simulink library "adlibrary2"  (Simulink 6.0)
settings: Solver=ode45  StartTime=0.0  StopTime=10.0  RelTol=1e-3
undefined symbols (not defined in the file or in its folder): adlibrary2, ADM, Bit, DDR, Generation, II, Location, Lower, SDRAM, SRAM, Width, XP, XPL, XRC, ZBT
libraries: xbsIndex_r3 x581, adlibrary2 x2
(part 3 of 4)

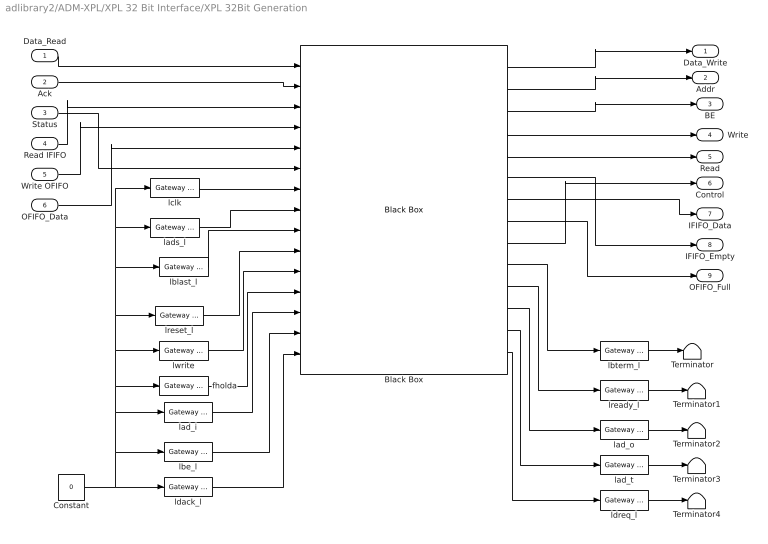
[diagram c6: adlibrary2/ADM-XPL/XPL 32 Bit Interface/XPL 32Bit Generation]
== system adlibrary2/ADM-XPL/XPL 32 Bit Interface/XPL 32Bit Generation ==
  Data_Read : Inport  Port=1  LatchInput=off
  Ack : Inport  Port=2  LatchInput=off
  Status : Inport  Port=3  LatchInput=off
  Read IFIFO : Inport  Port=4  LatchInput=off
  Write OFIFO : Inport  Port=5  LatchInput=off
  OFIFO_Data : Inport  Port=6  LatchInput=off
  Black Box : xbsIndex_r3/Black Box  init_code=lbif32_xpl_config  sim_method=Inactive  show_param=on
  Constant : Constant  Value=0
  Terminator{,1..4} (5 alike) : Terminator
  fholda : xbsIndex_r3/Gateway In  arith_type=Boolean  n_bits=8  bin_pt=6  quantization=Truncate  overflow=Wrap  period=1  timing_constraint=None  locs_specified=off  LOCs={}  needs_fixed_name=off  dbl_ovrd=off  show_param=off
  lad_i : xbsIndex_r3/Gateway In  arith_type=Unsigned  n_bits=64  bin_pt=0  quantization=Truncate  overflow=Wrap  period=1  timing_constraint=None  locs_specified=off  LOCs={}  needs_fixed_name=off  dbl_ovrd=off  show_param=off
  lad_o : xbsIndex_r3/Gateway Out  hdl_port=on  timing_constraint=None  locs_specified=off  LOCs={}  needs_fixed_name=off  show_param=off
  lad_t : xbsIndex_r3/Gateway Out  hdl_port=on  timing_constraint=None  locs_specified=off  LOCs={}  needs_fixed_name=off  show_param=off
  lads_l : xbsIndex_r3/Gateway In  arith_type=Boolean  n_bits=8  bin_pt=6  quantization=Truncate  overflow=Wrap  period=1  timing_constraint=None  locs_specified=off  LOCs={}  needs_fixed_name=off  dbl_ovrd=off  show_param=off
  lbe_l : xbsIndex_r3/Gateway In  arith_type=Unsigned  n_bits=8  bin_pt=0  quantization=Truncate  overflow=Wrap  period=1  timing_constraint=None  locs_specified=off  LOCs={}  needs_fixed_name=off  dbl_ovrd=off  show_param=off
  lblast_l : xbsIndex_r3/Gateway In  arith_type=Boolean  n_bits=8  bin_pt=6  quantization=Truncate  overflow=Wrap  period=1  timing_constraint=None  locs_specified=off  LOCs={}  needs_fixed_name=off  dbl_ovrd=off  show_param=off
  lbterm_l : xbsIndex_r3/Gateway Out  hdl_port=on  timing_constraint=None  locs_specified=off  LOCs={}  needs_fixed_name=off  show_param=off
  lclk : xbsIndex_r3/Gateway In  arith_type=Boolean  n_bits=8  bin_pt=6  quantization=Truncate  overflow=Wrap  period=1  timing_constraint=None  locs_specified=off  LOCs={}  needs_fixed_name=off  dbl_ovrd=off  show_param=off
  ldack_l : xbsIndex_r3/Gateway In  arith_type=Unsigned  n_bits=2  bin_pt=0  quantization=Truncate  overflow=Wrap  period=1  timing_constraint=None  locs_specified=off  LOCs={}  needs_fixed_name=off  dbl_ovrd=off  show_param=off
  ldreq_l : xbsIndex_r3/Gateway Out  hdl_port=on  timing_constraint=None  locs_specified=off  LOCs={}  needs_fixed_name=off  show_param=off
  lready_l : xbsIndex_r3/Gateway Out  hdl_port=on  timing_constraint=None  locs_specified=off  LOCs={}  needs_fixed_name=off  show_param=off
  lreset_l : xbsIndex_r3/Gateway In  arith_type=Boolean  n_bits=8  bin_pt=6  quantization=Truncate  overflow=Wrap  period=1  timing_constraint=None  locs_specified=off  LOCs={}  needs_fixed_name=off  dbl_ovrd=off  show_param=off
  lwrite : xbsIndex_r3/Gateway In  arith_type=Boolean  n_bits=8  bin_pt=6  quantization=Truncate  overflow=Wrap  period=1  timing_constraint=None  locs_specified=off  LOCs={}  needs_fixed_name=off  dbl_ovrd=off  show_param=off
  Data_Write : Outport
  Addr : Outport  Port=2
  BE : Outport  Port=3
  Write : Outport  Port=4
  Read : Outport  Port=5
  Control : Outport  Port=6
  IFIFO_Data : Outport  Port=7
  IFIFO_Empty : Outport  Port=8
  OFIFO_Full : Outport  Port=9
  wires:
  ldreq_l/1 -> Terminator4/1
  lad_t/1 -> Terminator3/1
  lad_o/1 -> Terminator2/1
  lready_l/1 -> Terminator1/1
  lbterm_l/1 -> Terminator/1
  Constant/1 -> lbe_l/1, lad_i/1, fholda/1, lwrite/1, lreset_l/1, lblast_l/1, lads_l/1, lclk/1, ldack_l/1
  ldack_l/1 -> Black Box/15
  lad_i/1 -> Black Box/13
  fholda/1 -> Black Box/12
  lwrite/1 -> Black Box/11
  lreset_l/1 -> Black Box/10
  lblast_l/1 -> Black Box/9
  lads_l/1 -> Black Box/8
  lclk/1 -> Black Box/7
  OFIFO_Data/1 -> Black Box/5
  Write OFIFO/1 -> Black Box/4
  Read IFIFO/1 -> Black Box/3
  Status/1 -> Black Box/6
  Ack/1 -> Black Box/2
  Data_Read/1 -> Black Box/1
  lbe_l/1 -> Black Box/14
  Black Box/1 -> Data_Write/1
  Black Box/2 -> Addr/1
  Black Box/3 -> BE/1
  Black Box/4 -> Write/1
  Black Box/5 -> Read/1
  Black Box/6 -> IFIFO_Empty/1
  Black Box/7 -> IFIFO_Data/1
  Black Box/8 -> OFIFO_Full/1
  Black Box/9 -> Control/1
  Black Box/10 -> lbterm_l/1
  Black Box/11 -> lready_l/1
  Black Box/12 -> lad_o/1
  Black Box/13 -> lad_t/1
  Black Box/14 -> ldreq_l/1

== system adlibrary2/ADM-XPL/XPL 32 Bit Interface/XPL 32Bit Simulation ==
  Data_Read : Inport  Port=1  LatchInput=off
  Ack : Inport  Port=2  LatchInput=off
  Status : Inport  Port=3  LatchInput=off
  Read IFIFO : Inport  Port=4  LatchInput=off
  Write OFIFO : Inport  Port=5  LatchInput=off
  OFIFO_Data : Inport  Port=6  LatchInput=off
  Disregard Subsystem : xbsIndex_r3/Disregard Subsystem  Tag=discardX
  Gateway Out{,1..5} (6 alike) : xbsIndex_r3/Gateway Out  hdl_port=off  timing_constraint=None  locs_specified=off  LOCs={}  needs_fixed_name=off  show_param=off
  S-Function : S-Function  FunctionName=lbif_plx32  Parameters=program,clock_ratio
  Subsystem : Subsystem
  Data_Write : Outport
  Addr : Outport  Port=2
  BE : Outport  Port=3
  Write : Outport  Port=4
  Read : Outport  Port=5
  Control : Outport  Port=6
  IFIFO_Data : Outport  Port=7
  IFIFO_Empty : Outport  Port=8
  OFIFO_Full : Outport  Port=9
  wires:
  Gateway Out5/1 -> S-Function/6
  Gateway Out4/1 -> S-Function/5
  Gateway Out3/1 -> S-Function/4
  Gateway Out2/1 -> S-Function/3
  Gateway Out1/1 -> S-Function/2
  Gateway Out/1 -> S-Function/1
  OFIFO_Data/1 -> Gateway Out5/1
  Write OFIFO/1 -> Gateway Out4/1
  Read IFIFO/1 -> Gateway Out3/1
  Status/1 -> Gateway Out2/1
  Ack/1 -> Gateway Out1/1
  Data_Read/1 -> Gateway Out/1
  S-Function/1 -> Subsystem/1(In1)
  S-Function/2 -> Subsystem/2(In2)
  S-Function/3 -> Subsystem/3(In9)
  S-Function/4 -> Subsystem/4(In3)
  S-Function/5 -> Subsystem/5(In4)
  S-Function/6 -> Subsystem/6(In5)
  S-Function/7 -> Subsystem/7(In6)
  S-Function/8 -> Subsystem/8(In7)
  Subsystem/1(Out1) -> Data_Write/1
  Subsystem/2(Out2) -> Addr/1
  Subsystem/9(Out8) -> OFIFO_Full/1
  Subsystem/8(Out7) -> IFIFO_Empty/1
  Subsystem/7(Out6) -> IFIFO_Data/1
  Subsystem/6(Out5) -> Control/1
  Subsystem/5(Out4) -> Read/1
  Subsystem/4(Out3) -> Write/1
  Subsystem/3(Out9) -> BE/1
  S-Function/9 -> Subsystem/9(In8)

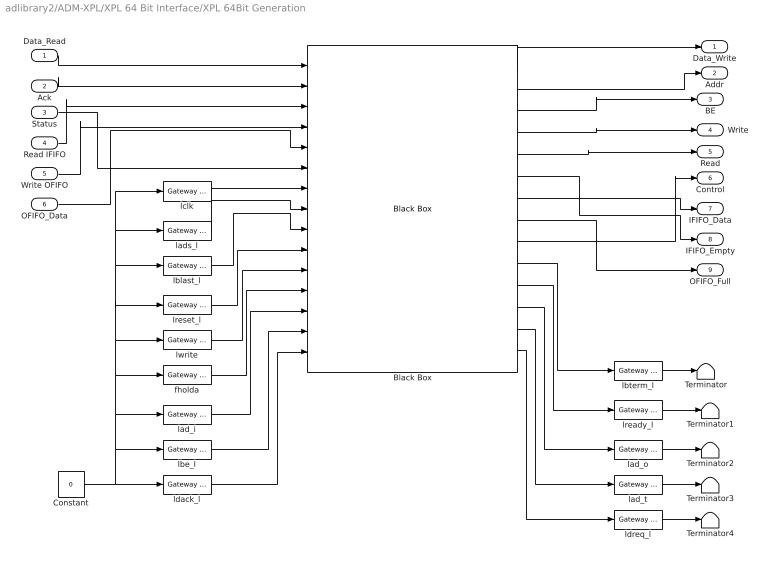
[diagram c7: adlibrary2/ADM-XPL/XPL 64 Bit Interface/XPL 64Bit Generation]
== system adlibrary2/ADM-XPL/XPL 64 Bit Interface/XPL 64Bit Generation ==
  Data_Read : Inport  Port=1  LatchInput=off
  Ack : Inport  Port=2  LatchInput=off
  Status : Inport  Port=3  LatchInput=off
  Read IFIFO : Inport  Port=4  LatchInput=off
  Write OFIFO : Inport  Port=5  LatchInput=off
  OFIFO_Data : Inport  Port=6  LatchInput=off
  Black Box : xbsIndex_r3/Black Box  init_code=lbif64_xpl_config  sim_method=Inactive  show_param=on
  Constant : Constant  Value=0
  Terminator{,1..4} (5 alike) : Terminator
  fholda : xbsIndex_r3/Gateway In  arith_type=Boolean  n_bits=8  bin_pt=6  quantization=Truncate  overflow=Wrap  period=1  timing_constraint=None  locs_specified=off  LOCs={}  needs_fixed_name=off  dbl_ovrd=off  show_param=off
  lad_i : xbsIndex_r3/Gateway In  arith_type=Unsigned  n_bits=64  bin_pt=0  quantization=Truncate  overflow=Wrap  period=1  timing_constraint=None  locs_specified=off  LOCs={}  needs_fixed_name=off  dbl_ovrd=off  show_param=off
  lad_o : xbsIndex_r3/Gateway Out  hdl_port=on  timing_constraint=None  locs_specified=off  LOCs={}  needs_fixed_name=off  show_param=off
  lad_t : xbsIndex_r3/Gateway Out  hdl_port=on  timing_constraint=None  locs_specified=off  LOCs={}  needs_fixed_name=off  show_param=off
  lads_l : xbsIndex_r3/Gateway In  arith_type=Boolean  n_bits=8  bin_pt=6  quantization=Truncate  overflow=Wrap  period=1  timing_constraint=None  locs_specified=off  LOCs={}  needs_fixed_name=off  dbl_ovrd=off  show_param=off
  lbe_l : xbsIndex_r3/Gateway In  arith_type=Unsigned  n_bits=8  bin_pt=0  quantization=Truncate  overflow=Wrap  period=1  timing_constraint=None  locs_specified=off  LOCs={}  needs_fixed_name=off  dbl_ovrd=off  show_param=off
  lblast_l : xbsIndex_r3/Gateway In  arith_type=Boolean  n_bits=8  bin_pt=6  quantization=Truncate  overflow=Wrap  period=1  timing_constraint=None  locs_specified=off  LOCs={}  needs_fixed_name=off  dbl_ovrd=off  show_param=off
  lbterm_l : xbsIndex_r3/Gateway Out  hdl_port=on  timing_constraint=None  locs_specified=off  LOCs={}  needs_fixed_name=off  show_param=off
  lclk : xbsIndex_r3/Gateway In  arith_type=Boolean  n_bits=8  bin_pt=6  quantization=Truncate  overflow=Wrap  period=1  timing_constraint=None  locs_specified=off  LOCs={}  needs_fixed_name=off  dbl_ovrd=off  show_param=off
  ldack_l : xbsIndex_r3/Gateway In  arith_type=Unsigned  n_bits=2  bin_pt=0  quantization=Truncate  overflow=Wrap  period=1  timing_constraint=None  locs_specified=off  LOCs={}  needs_fixed_name=off  dbl_ovrd=off  show_param=off
  ldreq_l : xbsIndex_r3/Gateway Out  hdl_port=on  timing_constraint=None  locs_specified=off  LOCs={}  needs_fixed_name=off  show_param=off
  lready_l : xbsIndex_r3/Gateway Out  hdl_port=on  timing_constraint=None  locs_specified=off  LOCs={}  needs_fixed_name=off  show_param=off
  lreset_l : xbsIndex_r3/Gateway In  arith_type=Boolean  n_bits=8  bin_pt=6  quantization=Truncate  overflow=Wrap  period=1  timing_constraint=None  locs_specified=off  LOCs={}  needs_fixed_name=off  dbl_ovrd=off  show_param=off
  lwrite : xbsIndex_r3/Gateway In  arith_type=Boolean  n_bits=8  bin_pt=6  quantization=Truncate  overflow=Wrap  period=1  timing_constraint=None  locs_specified=off  LOCs={}  needs_fixed_name=off  dbl_ovrd=off  show_param=off
  Data_Write : Outport
  Addr : Outport  Port=2
  BE : Outport  Port=3
  Write : Outport  Port=4
  Read : Outport  Port=5
  Control : Outport  Port=6
  IFIFO_Data : Outport  Port=7
  IFIFO_Empty : Outport  Port=8
  OFIFO_Full : Outport  Port=9
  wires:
  lbe_l/1 -> Black Box/14
  Data_Read/1 -> Black Box/1
  Ack/1 -> Black Box/2
  Status/1 -> Black Box/6
  Read IFIFO/1 -> Black Box/3
  Write OFIFO/1 -> Black Box/4
  OFIFO_Data/1 -> Black Box/5
  Black Box/1 -> Data_Write/1
  Black Box/2 -> Addr/1
  lclk/1 -> Black Box/7
  lads_l/1 -> Black Box/8
  lblast_l/1 -> Black Box/9
  lreset_l/1 -> Black Box/10
  lwrite/1 -> Black Box/11
  fholda/1 -> Black Box/12
  lad_i/1 -> Black Box/13
  ldack_l/1 -> Black Box/15
  Constant/1 -> ldack_l/1, lclk/1, lads_l/1, lblast_l/1, lreset_l/1, lwrite/1, fholda/1, lad_i/1, lbe_l/1
  lbterm_l/1 -> Terminator/1
  lready_l/1 -> Terminator1/1
  lad_o/1 -> Terminator2/1
  lad_t/1 -> Terminator3/1
  ldreq_l/1 -> Terminator4/1
  Black Box/14 -> ldreq_l/1
  Black Box/3 -> BE/1
  Black Box/4 -> Write/1
  Black Box/5 -> Read/1
  Black Box/6 -> IFIFO_Empty/1
  Black Box/7 -> IFIFO_Data/1
  Black Box/8 -> OFIFO_Full/1
  Black Box/9 -> Control/1
  Black Box/10 -> lbterm_l/1
  Black Box/11 -> lready_l/1
  Black Box/12 -> lad_o/1
  Black Box/13 -> lad_t/1

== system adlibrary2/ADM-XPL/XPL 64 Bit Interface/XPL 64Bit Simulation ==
  Data_Read : Inport  Port=1  LatchInput=off
  Ack : Inport  Port=2  LatchInput=off
  Status : Inport  Port=3  LatchInput=off
  Read IFIFO : Inport  Port=4  LatchInput=off
  Write OFIFO : Inport  Port=5  LatchInput=off
  OFIFO_Data : Inport  Port=6  LatchInput=off
  Disregard Subsystem : xbsIndex_r3/Disregard Subsystem  Tag=discardX
  Gateway Out{,1..8} (9 alike) : xbsIndex_r3/Gateway Out  hdl_port=off  timing_constraint=None  locs_specified=off  LOCs={}  needs_fixed_name=off  show_param=off
  S-Function : S-Function  FunctionName=lbif_xpl64  Parameters=program,clock_ratio
  Slice : xbsIndex_r3/Slice  mode=Lower Bit Location + Width  nbits=32  bit1=0  base1=MSB of Input  bit0=0  base0=LSB of Input  boolean_output=off  explicit_period=off  period=1  dbl_ovrd=off
  Slice1 : xbsIndex_r3/Slice  mode=Lower Bit Location + Width  nbits=32  bit1=0  base1=MSB of Input  bit0=32  base0=LSB of Input  boolean_output=off  explicit_period=off  period=1  dbl_ovrd=off
  Slice2 : xbsIndex_r3/Slice  mode=Lower Bit Location + Width  nbits=32  bit1=0  base1=MSB of Input  bit0=0  base0=LSB of Input  boolean_output=off  explicit_period=off  period=1  dbl_ovrd=off
  Slice3 : xbsIndex_r3/Slice  mode=Lower Bit Location + Width  nbits=32  bit1=0  base1=MSB of Input  bit0=32  base0=LSB of Input  boolean_output=off  explicit_period=off  period=1  dbl_ovrd=off
  Slice4 : xbsIndex_r3/Slice  mode=Lower Bit Location + Width  nbits=32  bit1=0  base1=MSB of Input  bit0=0  base0=LSB of Input  boolean_output=off  explicit_period=off  period=1  dbl_ovrd=off
  Slice5 : xbsIndex_r3/Slice  mode=Lower Bit Location + Width  nbits=32  bit1=0  base1=MSB of Input  bit0=32  base0=LSB of Input  boolean_output=off  explicit_period=off  period=1  dbl_ovrd=off
  Subsystem : Subsystem
  Data_Write : Outport
  Addr : Outport  Port=2
  BE : Outport  Port=3
  Write : Outport  Port=4
  Read : Outport  Port=5
  Control : Outport  Port=6
  IFIFO_Data : Outport  Port=7
  IFIFO_Empty : Outport  Port=8
  OFIFO_Full : Outport  Port=9
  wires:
  Data_Read/1 -> Slice/1, Slice1/1
  Ack/1 -> Gateway Out1/1
  Status/1 -> Slice2/1, Slice3/1
  Read IFIFO/1 -> Gateway Out3/1
  Write OFIFO/1 -> Gateway Out4/1
  OFIFO_Data/1 -> Slice4/1, Slice5/1
  Slice/1 -> Gateway Out/1
  Slice1/1 -> Gateway Out6/1
  Gateway Out/1 -> S-Function/1
  Gateway Out6/1 -> S-Function/2
  Gateway Out1/1 -> S-Function/3
  Slice2/1 -> Gateway Out2/1
  Slice3/1 -> Gateway Out7/1
  Gateway Out2/1 -> S-Function/4
  Gateway Out7/1 -> S-Function/5
  Gateway Out3/1 -> S-Function/6
  Gateway Out4/1 -> S-Function/7
  Slice4/1 -> Gateway Out5/1
  Slice5/1 -> Gateway Out8/1
  Gateway Out5/1 -> S-Function/8
  Gateway Out8/1 -> S-Function/9
  S-Function/1 -> Subsystem/1(data_write0)
  S-Function/2 -> Subsystem/2(data_write1)
  S-Function/3 -> Subsystem/3(addr)
  S-Function/4 -> Subsystem/4(be)
  S-Function/5 -> Subsystem/5(write)
  S-Function/6 -> Subsystem/6(read)
  S-Function/7 -> Subsystem/7(control0)
  S-Function/8 -> Subsystem/8(control1)
  S-Function/9 -> Subsystem/9(ififo_data0)
  S-Function/12 -> Subsystem/12(ofifo_full)
  S-Function/11 -> Subsystem/11(ififo_empty)
  S-Function/10 -> Subsystem/10(ififo_data1)
  Subsystem/9(Out9) -> OFIFO_Full/1
  Subsystem/8(Out8) -> IFIFO_Empty/1
  Subsystem/7(Out7) -> IFIFO_Data/1
  Subsystem/6(Out6) -> Control/1
  Subsystem/5(Out5) -> Read/1
  Subsystem/4(Out4) -> Write/1
  Subsystem/3(Out3) -> BE/1
  Subsystem/2(Out2) -> Addr/1
  Subsystem/1(Out1) -> Data_Write/1

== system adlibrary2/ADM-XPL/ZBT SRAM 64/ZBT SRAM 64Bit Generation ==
  d : Inport  Port=1  LatchInput=off
  a : Inport  Port=2  LatchInput=off
  w : Inport  Port=3  LatchInput=off
  r : Inport  Port=4  LatchInput=off
  be : Inport  Port=5  LatchInput=off
  Black Box : xbsIndex_r3/Black Box  init_code=zbt64_config  sim_method=Inactive  show_param=on
  Constant : Constant  Value=0
  Terminator{,1..3} (4 alike) : Terminator
  ra0 : xbsIndex_r3/Gateway Out  hdl_port=on  timing_constraint=None  locs_specified=off  LOCs={}  needs_fixed_name=off  show_param=off
  rc0 : xbsIndex_r3/Gateway Out  hdl_port=on  timing_constraint=None  locs_specified=off  LOCs={}  needs_fixed_name=off  show_param=off
  rd0_i : xbsIndex_r3/Gateway In  arith_type=Unsigned  n_bits=64  bin_pt=0  quantization=Truncate  overflow=Wrap  period=1  timing_constraint=None  locs_specified=off  LOCs={}  needs_fixed_name=off  dbl_ovrd=off  show_param=off
  rd0_o : xbsIndex_r3/Gateway Out  hdl_port=on  timing_constraint=None  locs_specified=off  LOCs={}  needs_fixed_name=off  show_param=off
  rd0_t : xbsIndex_r3/Gateway Out  hdl_port=on  timing_constraint=None  locs_specified=off  LOCs={}  needs_fixed_name=off  show_param=off
  q : Outport
  qv : Outport  Port=2
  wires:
  d/1 -> Black Box/1
  Black Box/1 -> q/1
  rd0_i/1 -> Black Box/6
  Constant/1 -> rd0_i/1
  rd0_o/1 -> Terminator/1
  rd0_t/1 -> Terminator1/1
  ra0/1 -> Terminator2/1
  rc0/1 -> Terminator3/1
  a/1 -> Black Box/2
  w/1 -> Black Box/3
  r/1 -> Black Box/4
  be/1 -> Black Box/5
  Black Box/2 -> qv/1
  Black Box/3 -> rd0_o/1
  Black Box/4 -> rd0_t/1
  Black Box/5 -> ra0/1
  Black Box/6 -> rc0/1

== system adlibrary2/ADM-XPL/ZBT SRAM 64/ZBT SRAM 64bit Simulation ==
  d : Inport  Port=1  LatchInput=off
  a : Inport  Port=2  LatchInput=off
  w : Inport  Port=3  LatchInput=off
  r : Inport  Port=4  LatchInput=off
  be : Inport  Port=5  LatchInput=off
  Concat : xbsIndex_r3/Concat  num_inputs=2  explicit_period=off  period=1  dbl_ovrd=off
  Disregard Subsystem : xbsIndex_r3/Disregard Subsystem  Tag=discardX
  Gateway In1 : xbsIndex_r3/Gateway In  arith_type=Unsigned  n_bits=32  bin_pt=0  quantization=Truncate  overflow=Wrap  period=1  timing_constraint=None  locs_specified=off  LOCs={}  needs_fixed_name=off  dbl_ovrd=on  show_param=off
  Gateway In6 : xbsIndex_r3/Gateway In  arith_type=Boolean  n_bits=1  bin_pt=0  quantization=Truncate  overflow=Wrap  period=1  timing_constraint=None  locs_specified=off  LOCs={}  needs_fixed_name=off  dbl_ovrd=on  show_param=off
  Gateway In7 : xbsIndex_r3/Gateway In  arith_type=Unsigned  n_bits=32  bin_pt=0  quantization=Truncate  overflow=Wrap  period=1  timing_constraint=None  locs_specified=off  LOCs={}  needs_fixed_name=off  dbl_ovrd=on  show_param=off
  Gateway Out{,1..5} (6 alike) : xbsIndex_r3/Gateway Out  hdl_port=off  timing_constraint=None  locs_specified=off  LOCs={}  needs_fixed_name=off  show_param=off
  S-Function : S-Function  FunctionName=zbt64
  Slice : xbsIndex_r3/Slice  mode=Lower Bit Location + Width  nbits=32  bit1=0  base1=MSB of Input  bit0=0  base0=LSB of Input  boolean_output=off  explicit_period=off  period=1  dbl_ovrd=off
  Slice1 : xbsIndex_r3/Slice  mode=Lower Bit Location + Width  nbits=32  bit1=0  base1=MSB of Input  bit0=32  base0=LSB of Input  boolean_output=off  explicit_period=off  period=1  dbl_ovrd=off
  q : Outport
  qv : Outport  Port=2
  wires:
  a/1 -> Gateway Out2/1
  w/1 -> Gateway Out3/1
  S-Function/1 -> Gateway In7/1
  Gateway Out/1 -> S-Function/1
  Gateway Out1/1 -> S-Function/2
  Gateway Out2/1 -> S-Function/3
  Gateway Out3/1 -> S-Function/4
  r/1 -> Gateway Out4/1
  Gateway Out4/1 -> S-Function/5
  S-Function/2 -> Gateway In1/1
  Gateway In6/1 -> qv/1
  S-Function/3 -> Gateway In6/1
  be/1 -> Gateway Out5/1
  Gateway Out5/1 -> S-Function/6
  Slice1/1 -> Gateway Out/1
  Slice/1 -> Gateway Out1/1
  d/1 -> Slice1/1, Slice/1
  Gateway In7/1 -> Concat/1
  Gateway In1/1 -> Concat/2
  Concat/1 -> q/1

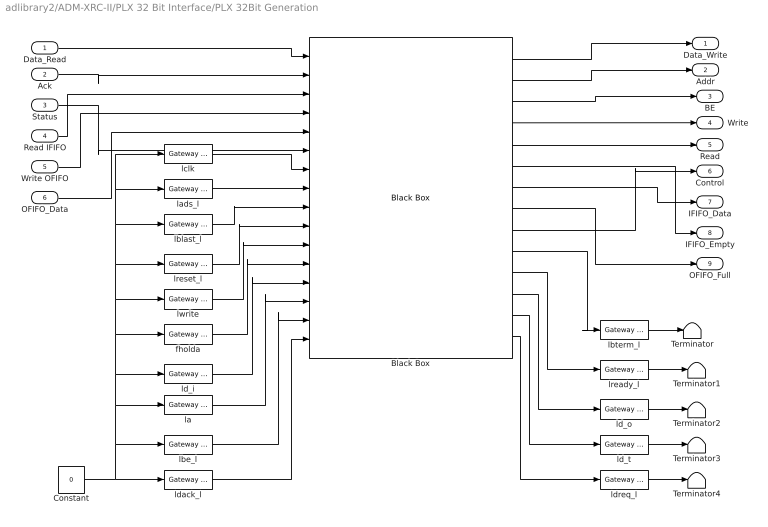
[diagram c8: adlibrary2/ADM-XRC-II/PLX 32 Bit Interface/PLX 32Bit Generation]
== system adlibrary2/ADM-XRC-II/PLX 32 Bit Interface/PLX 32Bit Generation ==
  Data_Read : Inport  Port=1  LatchInput=off
  Ack : Inport  Port=2  LatchInput=off
  Status : Inport  Port=3  LatchInput=off
  Read IFIFO : Inport  Port=4  LatchInput=off
  Write OFIFO : Inport  Port=5  LatchInput=off
  OFIFO_Data : Inport  Port=6  LatchInput=off
  Black Box : xbsIndex_r3/Black Box  init_code=lbif32_plx_config  sim_method=Inactive  show_param=on
  Constant : Constant  Value=0
  Terminator{,1..4} (5 alike) : Terminator
  fholda : xbsIndex_r3/Gateway In  arith_type=Boolean  n_bits=8  bin_pt=6  quantization=Truncate  overflow=Wrap  period=1  timing_constraint=None  locs_specified=off  LOCs={}  needs_fixed_name=off  dbl_ovrd=off  show_param=off
  la : xbsIndex_r3/Gateway In  arith_type=Unsigned  n_bits=24  bin_pt=0  quantization=Truncate  overflow=Wrap  period=1  timing_constraint=None  locs_specified=off  LOCs={}  needs_fixed_name=off  dbl_ovrd=off  show_param=off
  lads_l : xbsIndex_r3/Gateway In  arith_type=Boolean  n_bits=8  bin_pt=6  quantization=Truncate  overflow=Wrap  period=1  timing_constraint=None  locs_specified=off  LOCs={}  needs_fixed_name=off  dbl_ovrd=off  show_param=off
  lbe_l : xbsIndex_r3/Gateway In  arith_type=Unsigned  n_bits=4  bin_pt=0  quantization=Truncate  overflow=Wrap  period=1  timing_constraint=None  locs_specified=off  LOCs={}  needs_fixed_name=off  dbl_ovrd=off  show_param=off
  lblast_l : xbsIndex_r3/Gateway In  arith_type=Boolean  n_bits=8  bin_pt=6  quantization=Truncate  overflow=Wrap  period=1  timing_constraint=None  locs_specified=off  LOCs={}  needs_fixed_name=off  dbl_ovrd=off  show_param=off
  lbterm_l : xbsIndex_r3/Gateway Out  hdl_port=on  timing_constraint=None  locs_specified=off  LOCs={}  needs_fixed_name=off  show_param=off
  lclk : xbsIndex_r3/Gateway In  arith_type=Boolean  n_bits=8  bin_pt=6  quantization=Truncate  overflow=Wrap  period=1  timing_constraint=None  locs_specified=off  LOCs={}  needs_fixed_name=off  dbl_ovrd=off  show_param=off
  ld_i : xbsIndex_r3/Gateway In  arith_type=Unsigned  n_bits=32  bin_pt=0  quantization=Truncate  overflow=Wrap  period=1  timing_constraint=None  locs_specified=off  LOCs={}  needs_fixed_name=off  dbl_ovrd=off  show_param=off
  ld_o : xbsIndex_r3/Gateway Out  hdl_port=on  timing_constraint=None  locs_specified=off  LOCs={}  needs_fixed_name=off  show_param=off
  ld_t : xbsIndex_r3/Gateway Out  hdl_port=on  timing_constraint=None  locs_specified=off  LOCs={}  needs_fixed_name=off  show_param=off
  ldack_l : xbsIndex_r3/Gateway In  arith_type=Unsigned  n_bits=2  bin_pt=0  quantization=Truncate  overflow=Wrap  period=1  timing_constraint=None  locs_specified=off  LOCs={}  needs_fixed_name=off  dbl_ovrd=off  show_param=off
  ldreq_l : xbsIndex_r3/Gateway Out  hdl_port=on  timing_constraint=None  locs_specified=off  LOCs={}  needs_fixed_name=off  show_param=off
  lready_l : xbsIndex_r3/Gateway Out  hdl_port=on  timing_constraint=None  locs_specified=off  LOCs={}  needs_fixed_name=off  show_param=off
  lreset_l : xbsIndex_r3/Gateway In  arith_type=Boolean  n_bits=8  bin_pt=6  quantization=Truncate  overflow=Wrap  period=1  timing_constraint=None  locs_specified=off  LOCs={}  needs_fixed_name=off  dbl_ovrd=off  show_param=off
  lwrite : xbsIndex_r3/Gateway In  arith_type=Boolean  n_bits=8  bin_pt=6  quantization=Truncate  overflow=Wrap  period=1  timing_constraint=None  locs_specified=off  LOCs={}  needs_fixed_name=off  dbl_ovrd=off  show_param=off
  Data_Write : Outport
  Addr : Outport  Port=2
  BE : Outport  Port=3
  Write : Outport  Port=4
  Read : Outport  Port=5
  Control : Outport  Port=6
  IFIFO_Data : Outport  Port=7
  IFIFO_Empty : Outport  Port=8
  OFIFO_Full : Outport  Port=9
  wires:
  Data_Read/1 -> Black Box/1
  Ack/1 -> Black Box/2
  Status/1 -> Black Box/6
  Read IFIFO/1 -> Black Box/3
  Write OFIFO/1 -> Black Box/4
  OFIFO_Data/1 -> Black Box/5
  lclk/1 -> Black Box/7
  lads_l/1 -> Black Box/8
  lblast_l/1 -> Black Box/9
  lreset_l/1 -> Black Box/10
  lwrite/1 -> Black Box/11
  fholda/1 -> Black Box/12
  ld_i/1 -> Black Box/13
  la/1 -> Black Box/14
  lbe_l/1 -> Black Box/15
  ldack_l/1 -> Black Box/16
  Constant/1 -> ldack_l/1, lclk/1, lads_l/1, lblast_l/1, lreset_l/1, lwrite/1, fholda/1, ld_i/1, la/1, lbe_l/1
  lbterm_l/1 -> Terminator/1
  lready_l/1 -> Terminator1/1
  ld_o/1 -> Terminator2/1
  ld_t/1 -> Terminator3/1
  ldreq_l/1 -> Terminator4/1
  Black Box/1 -> Data_Write/1
  Black Box/2 -> Addr/1
  Black Box/3 -> BE/1
  Black Box/4 -> Write/1
  Black Box/5 -> Read/1
  Black Box/7 -> IFIFO_Data/1
  Black Box/8 -> OFIFO_Full/1
  Black Box/6 -> IFIFO_Empty/1
  Black Box/9 -> Control/1
  Black Box/10 -> lbterm_l/1
  Black Box/11 -> lready_l/1
  Black Box/12 -> ld_o/1
  Black Box/13 -> ld_t/1
  Black Box/14 -> ldreq_l/1

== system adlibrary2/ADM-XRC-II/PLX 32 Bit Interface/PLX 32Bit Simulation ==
  Data_Read : Inport  Port=1  LatchInput=off
  Ack : Inport  Port=2  LatchInput=off
  Status : Inport  Port=3  LatchInput=off
  Read IFIFO : Inport  Port=4  LatchInput=off
  Write OFIFO : Inport  Port=5  LatchInput=off
  OFIFO_Data : Inport  Port=6  LatchInput=off
  Disregard Subsystem : xbsIndex_r3/Disregard Subsystem  Tag=discardX
  Gateway Out{,1..5} (6 alike) : xbsIndex_r3/Gateway Out  hdl_port=off  timing_constraint=None  locs_specified=off  LOCs={}  needs_fixed_name=off  show_param=off
  S-Function : S-Function  FunctionName=lbif_plx32  Parameters=program,clock_ratio
  Subsystem : Subsystem
  Data_Write : Outport
  Addr : Outport  Port=2
  BE : Outport  Port=3
  Write : Outport  Port=4
  Read : Outport  Port=5
  Control : Outport  Port=6
  IFIFO_Data : Outport  Port=7
  IFIFO_Empty : Outport  Port=8
  OFIFO_Full : Outport  Port=9
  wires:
  Subsystem/2(Out2) -> Addr/1
  Subsystem/1(Out1) -> Data_Write/1
  S-Function/2 -> Subsystem/2(In2)
  S-Function/1 -> Subsystem/1(In1)
  Gateway Out5/1 -> S-Function/6
  Gateway Out4/1 -> S-Function/5
  Gateway Out3/1 -> S-Function/4
  Gateway Out2/1 -> S-Function/3
  Gateway Out1/1 -> S-Function/2
  Gateway Out/1 -> S-Function/1
  OFIFO_Data/1 -> Gateway Out5/1
  Write OFIFO/1 -> Gateway Out4/1
  Read IFIFO/1 -> Gateway Out3/1
  Status/1 -> Gateway Out2/1
  Ack/1 -> Gateway Out1/1
  Data_Read/1 -> Gateway Out/1
  S-Function/3 -> Subsystem/3(In9)
  Subsystem/3(Out9) -> BE/1
  S-Function/4 -> Subsystem/4(In3)
  S-Function/5 -> Subsystem/5(In4)
  S-Function/6 -> Subsystem/6(In5)
  S-Function/7 -> Subsystem/7(In6)
  S-Function/8 -> Subsystem/8(In7)
  S-Function/9 -> Subsystem/9(In8)
  Subsystem/4(Out3) -> Write/1
  Subsystem/5(Out4) -> Read/1
  Subsystem/6(Out5) -> Control/1
  Subsystem/7(Out6) -> IFIFO_Data/1
  Subsystem/8(Out7) -> IFIFO_Empty/1
  Subsystem/9(Out8) -> OFIFO_Full/1

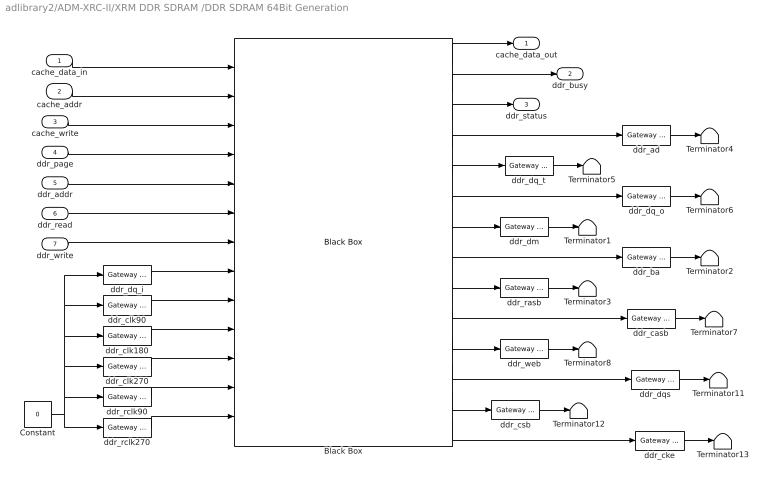
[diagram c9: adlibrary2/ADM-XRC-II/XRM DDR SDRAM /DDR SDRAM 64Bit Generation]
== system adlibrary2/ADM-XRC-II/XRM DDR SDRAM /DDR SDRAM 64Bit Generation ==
  cache_data_in : Inport  Port=1  LatchInput=off
  cache_addr : Inport  Port=2  LatchInput=off
  cache_write : Inport  Port=3  LatchInput=off
  ddr_page : Inport  Port=4  LatchInput=off
  ddr_addr : Inport  Port=5  LatchInput=off
  ddr_read : Inport  Port=6  LatchInput=off
  ddr_write : Inport  Port=7  LatchInput=off
  Black Box : xbsIndex_r3/Black Box  init_code=ddr64_config  sim_method=Inactive  show_param=on
  Constant : Constant  Value=0
  Terminator{1..8,11..13} (11 alike) : Terminator
  ddr_ad : xbsIndex_r3/Gateway Out  hdl_port=on  timing_constraint=None  locs_specified=off  LOCs={}  needs_fixed_name=off  show_param=off
  ddr_ba : xbsIndex_r3/Gateway Out  hdl_port=on  timing_constraint=None  locs_specified=off  LOCs={}  needs_fixed_name=off  show_param=off
  ddr_casb : xbsIndex_r3/Gateway Out  hdl_port=on  timing_constraint=None  locs_specified=off  LOCs={}  needs_fixed_name=off  show_param=off
  ddr_cke : xbsIndex_r3/Gateway Out  hdl_port=on  timing_constraint=None  locs_specified=off  LOCs={}  needs_fixed_name=off  show_param=off
  ddr_clk180 : xbsIndex_r3/Gateway In  arith_type=Boolean  n_bits=64  bin_pt=0  quantization=Truncate  overflow=Wrap  period=1  timing_constraint=None  locs_specified=off  LOCs={}  needs_fixed_name=off  dbl_ovrd=off  show_param=off
  ddr_clk270 : xbsIndex_r3/Gateway In  arith_type=Boolean  n_bits=64  bin_pt=0  quantization=Truncate  overflow=Wrap  period=1  timing_constraint=None  locs_specified=off  LOCs={}  needs_fixed_name=off  dbl_ovrd=off  show_param=off
  ddr_clk90 : xbsIndex_r3/Gateway In  arith_type=Boolean  n_bits=64  bin_pt=0  quantization=Truncate  overflow=Wrap  period=1  timing_constraint=None  locs_specified=off  LOCs={}  needs_fixed_name=off  dbl_ovrd=off  show_param=off
  ddr_csb : xbsIndex_r3/Gateway Out  hdl_port=on  timing_constraint=None  locs_specified=off  LOCs={}  needs_fixed_name=off  show_param=off
  ddr_dm : xbsIndex_r3/Gateway Out  hdl_port=on  timing_constraint=None  locs_specified=off  LOCs={}  needs_fixed_name=off  show_param=off
  ddr_dq_i : xbsIndex_r3/Gateway In  arith_type=Unsigned  n_bits=64  bin_pt=0  quantization=Truncate  overflow=Wrap  period=1  timing_constraint=None  locs_specified=off  LOCs={}  needs_fixed_name=off  dbl_ovrd=off  show_param=off
  ddr_dq_o : xbsIndex_r3/Gateway Out  hdl_port=on  timing_constraint=None  locs_specified=off  LOCs={}  needs_fixed_name=off  show_param=off
  ddr_dq_t : xbsIndex_r3/Gateway Out  hdl_port=on  timing_constraint=None  locs_specified=off  LOCs={}  needs_fixed_name=off  show_param=off
  ddr_dqs : xbsIndex_r3/Gateway Out  hdl_port=on  timing_constraint=None  locs_specified=off  LOCs={}  needs_fixed_name=off  show_param=off
  ddr_rasb : xbsIndex_r3/Gateway Out  hdl_port=on  timing_constraint=None  locs_specified=off  LOCs={}  needs_fixed_name=off  show_param=off
  ddr_rclk270 : xbsIndex_r3/Gateway In  arith_type=Boolean  n_bits=64  bin_pt=0  quantization=Truncate  overflow=Wrap  period=1  timing_constraint=None  locs_specified=off  LOCs={}  needs_fixed_name=off  dbl_ovrd=off  show_param=off
  ddr_rclk90 : xbsIndex_r3/Gateway In  arith_type=Boolean  n_bits=64  bin_pt=0  quantization=Truncate  overflow=Wrap  period=1  timing_constraint=None  locs_specified=off  LOCs={}  needs_fixed_name=off  dbl_ovrd=off  show_param=off
  ddr_web : xbsIndex_r3/Gateway Out  hdl_port=on  timing_constraint=None  locs_specified=off  LOCs={}  needs_fixed_name=off  show_param=off
  cache_data_out : Outport
  ddr_busy : Outport  Port=2
  ddr_status : Outport  Port=3
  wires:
  Constant/1 -> ddr_clk90/1, ddr_dq_i/1, ddr_clk180/1, ddr_clk270/1, ddr_rclk90/1, ddr_rclk270/1
  ddr_clk90/1 -> Black Box/9
  ddr_dq_i/1 -> Black Box/8
  cache_data_in/1 -> Black Box/1
  cache_addr/1 -> Black Box/2
  cache_write/1 -> Black Box/3
  ddr_page/1 -> Black Box/4
  ddr_addr/1 -> Black Box/5
  ddr_read/1 -> Black Box/6
  ddr_write/1 -> Black Box/7
  Black Box/1 -> cache_data_out/1
  Black Box/2 -> ddr_busy/1
  Black Box/3 -> ddr_status/1
  Black Box/4 -> ddr_ad/1
  ddr_ad/1 -> Terminator4/1
  ddr_dq_t/1 -> Terminator5/1
  Black Box/5 -> ddr_dq_t/1
  ddr_dq_o/1 -> Terminator6/1
  Black Box/6 -> ddr_dq_o/1
  ddr_dm/1 -> Terminator1/1
  Black Box/7 -> ddr_dm/1
  ddr_ba/1 -> Terminator2/1
  Black Box/8 -> ddr_ba/1
  ddr_rasb/1 -> Terminator3/1
  Black Box/9 -> ddr_rasb/1
  ddr_casb/1 -> Terminator7/1
  Black Box/10 -> ddr_casb/1
  ddr_web/1 -> Terminator8/1
  Black Box/11 -> ddr_web/1
  ddr_dqs/1 -> Terminator11/1
  ddr_csb/1 -> Terminator12/1
  Black Box/13 -> ddr_csb/1
  ddr_cke/1 -> Terminator13/1
  Black Box/14 -> ddr_cke/1
  ddr_clk180/1 -> Black Box/10
  ddr_clk270/1 -> Black Box/11
  ddr_rclk90/1 -> Black Box/12
  ddr_rclk270/1 -> Black Box/13
  Black Box/12 -> ddr_dqs/1

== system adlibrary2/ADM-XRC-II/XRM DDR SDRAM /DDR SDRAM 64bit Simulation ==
  cache_data_in : Inport  Port=1  LatchInput=off
  cache_addr : Inport  Port=2  LatchInput=off
  cache_write : Inport  Port=3  LatchInput=off
  ddr_page : Inport  Port=4  LatchInput=off
  ddr_addr : Inport  Port=5  LatchInput=off
  ddr_read : Inport  Port=6  LatchInput=off
  ddr_write : Inport  Port=7  LatchInput=off
  Disregard Subsystem : xbsIndex_r3/Disregard Subsystem  Tag=discardX
  S-Function : S-Function  FunctionName=ddr64  Parameters=memsize
  Subsystem : Subsystem
  gi{0..6} (7 alike) : xbsIndex_r3/Gateway Out  hdl_port=off  timing_constraint=None  locs_specified=off  LOCs={}  needs_fixed_name=off  show_param=off
  cache_data_out : Outport
  ddr_busy : Outport  Port=2
  ddr_status : Outport  Port=3
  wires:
  S-Function/1 -> Subsystem/1(In1)
  S-Function/2 -> Subsystem/2(In2)
  cache_data_in/1 -> gi0/1
  cache_addr/1 -> gi1/1
  cache_write/1 -> gi2/1
  ddr_page/1 -> gi3/1
  ddr_addr/1 -> gi4/1
  ddr_read/1 -> gi5/1
  ddr_write/1 -> gi6/1
  gi0/1 -> S-Function/1
  gi1/1 -> S-Function/2
  gi2/1 -> S-Function/3
  gi3/1 -> S-Function/4
  gi4/1 -> S-Function/5
  gi5/1 -> S-Function/6
  gi6/1 -> S-Function/7
  S-Function/3 -> Subsystem/3(In3)
  Subsystem/1(Out1) -> cache_data_out/1
  Subsystem/2(Out2) -> ddr_busy/1
  Subsystem/3(Out3) -> ddr_status/1

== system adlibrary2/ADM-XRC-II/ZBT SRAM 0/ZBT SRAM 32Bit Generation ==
  d : Inport  Port=1  LatchInput=off
  a : Inport  Port=2  LatchInput=off
  w : Inport  Port=3  LatchInput=off
  r : Inport  Port=4  LatchInput=off
  be : Inport  Port=5  LatchInput=off
  Black Box : xbsIndex_r3/Black Box  init_code=zbt32_config  sim_method=Inactive  show_param=on
  Constant : Constant  Value=0
  Terminator{,1..3} (4 alike) : Terminator
  ra0 : xbsIndex_r3/Gateway Out  hdl_port=on  timing_constraint=None  locs_specified=off  LOCs={}  needs_fixed_name=off  show_param=off
  rc0 : xbsIndex_r3/Gateway Out  hdl_port=on  timing_constraint=None  locs_specified=off  LOCs={}  needs_fixed_name=off  show_param=off
  rd0_i : xbsIndex_r3/Gateway In  arith_type=Unsigned  n_bits=32  bin_pt=0  quantization=Truncate  overflow=Wrap  period=1  timing_constraint=None  locs_specified=off  LOCs={}  needs_fixed_name=off  dbl_ovrd=off  show_param=off
  rd0_o : xbsIndex_r3/Gateway Out  hdl_port=on  timing_constraint=None  locs_specified=off  LOCs={}  needs_fixed_name=off  show_param=off
  rd0_t : xbsIndex_r3/Gateway Out  hdl_port=on  timing_constraint=None  locs_specified=off  LOCs={}  needs_fixed_name=off  show_param=off
  q : Outport
  qv : Outport  Port=2
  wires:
  Black Box/6 -> rc0/1
  Black Box/5 -> ra0/1
  Black Box/4 -> rd0_t/1
  Black Box/3 -> rd0_o/1
  r/1 -> Black Box/4
  w/1 -> Black Box/3
  a/1 -> Black Box/2
  rc0/1 -> Terminator3/1
  ra0/1 -> Terminator2/1
  rd0_t/1 -> Terminator1/1
  rd0_o/1 -> Terminator/1
  Constant/1 -> rd0_i/1
  Black Box/2 -> qv/1
  Black Box/1 -> q/1
  d/1 -> Black Box/1
  rd0_i/1 -> Black Box/6
  be/1 -> Black Box/5

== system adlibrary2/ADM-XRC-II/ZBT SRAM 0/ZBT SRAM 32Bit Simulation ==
  d : Inport  Port=1  LatchInput=off
  a : Inport  Port=2  LatchInput=off
  w : Inport  Port=3  LatchInput=off
  r : Inport  Port=4  LatchInput=off
  be : Inport  Port=5  LatchInput=off
  Disregard Subsystem : xbsIndex_r3/Disregard Subsystem  Tag=discardX
  Gateway In6 : xbsIndex_r3/Gateway In  arith_type=Boolean  n_bits=1  bin_pt=0  quantization=Truncate  overflow=Wrap  period=1  timing_constraint=None  locs_specified=off  LOCs={}  needs_fixed_name=off  dbl_ovrd=on  show_param=off
  Gateway In7 : xbsIndex_r3/Gateway In  arith_type=Unsigned  n_bits=32  bin_pt=0  quantization=Truncate  overflow=Wrap  period=1  timing_constraint=None  locs_specified=off  LOCs={}  needs_fixed_name=off  dbl_ovrd=on  show_param=off
  Gateway Out{,1..4} (5 alike) : xbsIndex_r3/Gateway Out  hdl_port=off  timing_constraint=None  locs_specified=off  LOCs={}  needs_fixed_name=off  show_param=off
  S-Function : S-Function  FunctionName=zbt32
  q : Outport
  qv : Outport  Port=2
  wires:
  S-Function/2 -> Gateway In6/1
  Gateway In7/1 -> q/1
  Gateway In6/1 -> qv/1
  Gateway Out3/1 -> S-Function/4
  Gateway Out2/1 -> S-Function/3
  Gateway Out1/1 -> S-Function/2
  Gateway Out/1 -> S-Function/1
  S-Function/1 -> Gateway In7/1
  r/1 -> Gateway Out3/1
  w/1 -> Gateway Out2/1
  a/1 -> Gateway Out1/1
  d/1 -> Gateway Out/1
  Gateway Out4/1 -> S-Function/5
  be/1 -> Gateway Out4/1

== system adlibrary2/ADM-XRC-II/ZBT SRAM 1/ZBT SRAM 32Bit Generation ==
  d : Inport  Port=1  LatchInput=off
  a : Inport  Port=2  LatchInput=off
  w : Inport  Port=3  LatchInput=off
  r : Inport  Port=4  LatchInput=off
  be : Inport  Port=5  LatchInput=off
  Black Box : xbsIndex_r3/Black Box  init_code=zbt32_config  sim_method=Inactive  show_param=on
  Constant : Constant  Value=0
  Terminator{,1..3} (4 alike) : Terminator
  ra1 : xbsIndex_r3/Gateway Out  hdl_port=on  timing_constraint=None  locs_specified=off  LOCs={}  needs_fixed_name=off  show_param=off
  rc1 : xbsIndex_r3/Gateway Out  hdl_port=on  timing_constraint=None  locs_specified=off  LOCs={}  needs_fixed_name=off  show_param=off
  rd1_i : xbsIndex_r3/Gateway In  arith_type=Unsigned  n_bits=32  bin_pt=0  quantization=Truncate  overflow=Wrap  period=1  timing_constraint=None  locs_specified=off  LOCs={}  needs_fixed_name=off  dbl_ovrd=off  show_param=off
  rd1_o : xbsIndex_r3/Gateway Out  hdl_port=on  timing_constraint=None  locs_specified=off  LOCs={}  needs_fixed_name=off  show_param=off
  rd1_t : xbsIndex_r3/Gateway Out  hdl_port=on  timing_constraint=None  locs_specified=off  LOCs={}  needs_fixed_name=off  show_param=off
  q : Outport
  qv : Outport  Port=2
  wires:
  Black Box/6 -> rc1/1
  Black Box/5 -> ra1/1
  Black Box/4 -> rd1_t/1
  Black Box/3 -> rd1_o/1
  r/1 -> Black Box/4
  w/1 -> Black Box/3
  a/1 -> Black Box/2
  rc1/1 -> Terminator3/1
  ra1/1 -> Terminator2/1
  rd1_t/1 -> Terminator1/1
  rd1_o/1 -> Terminator/1
  Constant/1 -> rd1_i/1
  Black Box/2 -> qv/1
  Black Box/1 -> q/1
  d/1 -> Black Box/1
  rd1_i/1 -> Black Box/6
  be/1 -> Black Box/5

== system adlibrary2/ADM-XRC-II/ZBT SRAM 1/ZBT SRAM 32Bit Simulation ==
  d : Inport  Port=1  LatchInput=off
  a : Inport  Port=2  LatchInput=off
  w : Inport  Port=3  LatchInput=off
  r : Inport  Port=4  LatchInput=off
  be : Inport  Port=5  LatchInput=off
  Disregard Subsystem : xbsIndex_r3/Disregard Subsystem  Tag=discardX
  Gateway In6 : xbsIndex_r3/Gateway In  arith_type=Boolean  n_bits=1  bin_pt=0  quantization=Truncate  overflow=Wrap  period=1  timing_constraint=None  locs_specified=off  LOCs={}  needs_fixed_name=off  dbl_ovrd=on  show_param=off
  Gateway In7 : xbsIndex_r3/Gateway In  arith_type=Unsigned  n_bits=32  bin_pt=0  quantization=Truncate  overflow=Wrap  period=1  timing_constraint=None  locs_specified=off  LOCs={}  needs_fixed_name=off  dbl_ovrd=on  show_param=off
  Gateway Out{,1..4} (5 alike) : xbsIndex_r3/Gateway Out  hdl_port=off  timing_constraint=None  locs_specified=off  LOCs={}  needs_fixed_name=off  show_param=off
  S-Function : S-Function  FunctionName=zbt32
  q : Outport
  qv : Outport  Port=2
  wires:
  S-Function/2 -> Gateway In6/1
  Gateway In7/1 -> q/1
  Gateway In6/1 -> qv/1
  Gateway Out3/1 -> S-Function/4
  Gateway Out2/1 -> S-Function/3
  Gateway Out1/1 -> S-Function/2
  Gateway Out/1 -> S-Function/1
  S-Function/1 -> Gateway In7/1
  r/1 -> Gateway Out3/1
  w/1 -> Gateway Out2/1
  a/1 -> Gateway Out1/1
  d/1 -> Gateway Out/1
  Gateway Out4/1 -> S-Function/5
  be/1 -> Gateway Out4/1

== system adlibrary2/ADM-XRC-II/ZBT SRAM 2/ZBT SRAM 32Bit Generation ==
  d : Inport  Port=1  LatchInput=off
  a : Inport  Port=2  LatchInput=off
  w : Inport  Port=3  LatchInput=off
  r : Inport  Port=4  LatchInput=off
  be : Inport  Port=5  LatchInput=off
  Black Box : xbsIndex_r3/Black Box  init_code=zbt32_config  sim_method=Inactive  show_param=on
  Constant : Constant  Value=0
  Terminator{,1..3} (4 alike) : Terminator
  ra2 : xbsIndex_r3/Gateway Out  hdl_port=on  timing_constraint=None  locs_specified=off  LOCs={}  needs_fixed_name=off  show_param=off
  rc2 : xbsIndex_r3/Gateway Out  hdl_port=on  timing_constraint=None  locs_specified=off  LOCs={}  needs_fixed_name=off  show_param=off
  rd2_i : xbsIndex_r3/Gateway In  arith_type=Unsigned  n_bits=32  bin_pt=0  quantization=Truncate  overflow=Wrap  period=1  timing_constraint=None  locs_specified=off  LOCs={}  needs_fixed_name=off  dbl_ovrd=off  show_param=off
  rd2_o : xbsIndex_r3/Gateway Out  hdl_port=on  timing_constraint=None  locs_specified=off  LOCs={}  needs_fixed_name=off  show_param=off
  rd2_t : xbsIndex_r3/Gateway Out  hdl_port=on  timing_constraint=None  locs_specified=off  LOCs={}  needs_fixed_name=off  show_param=off
  q : Outport
  qv : Outport  Port=2
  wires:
  Black Box/6 -> rc2/1
  Black Box/5 -> ra2/1
  Black Box/4 -> rd2_t/1
  Black Box/3 -> rd2_o/1
  r/1 -> Black Box/4
  w/1 -> Black Box/3
  a/1 -> Black Box/2
  rc2/1 -> Terminator3/1
  ra2/1 -> Terminator2/1
  rd2_t/1 -> Terminator1/1
  rd2_o/1 -> Terminator/1
  Constant/1 -> rd2_i/1
  Black Box/2 -> qv/1
  Black Box/1 -> q/1
  d/1 -> Black Box/1
  rd2_i/1 -> Black Box/6
  be/1 -> Black Box/5

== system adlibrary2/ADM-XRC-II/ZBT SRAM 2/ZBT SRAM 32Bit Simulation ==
  d : Inport  Port=1  LatchInput=off
  a : Inport  Port=2  LatchInput=off
  w : Inport  Port=3  LatchInput=off
  r : Inport  Port=4  LatchInput=off
  be : Inport  Port=5  LatchInput=off
  Disregard Subsystem : xbsIndex_r3/Disregard Subsystem  Tag=discardX
  Gateway In6 : xbsIndex_r3/Gateway In  arith_type=Boolean  n_bits=1  bin_pt=0  quantization=Truncate  overflow=Wrap  period=1  timing_constraint=None  locs_specified=off  LOCs={}  needs_fixed_name=off  dbl_ovrd=on  show_param=off
  Gateway In7 : xbsIndex_r3/Gateway In  arith_type=Unsigned  n_bits=32  bin_pt=0  quantization=Truncate  overflow=Wrap  period=1  timing_constraint=None  locs_specified=off  LOCs={}  needs_fixed_name=off  dbl_ovrd=on  show_param=off
  Gateway Out{,1..4} (5 alike) : xbsIndex_r3/Gateway Out  hdl_port=off  timing_constraint=None  locs_specified=off  LOCs={}  needs_fixed_name=off  show_param=off
  S-Function : S-Function  FunctionName=zbt32
  q : Outport
  qv : Outport  Port=2
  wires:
  S-Function/2 -> Gateway In6/1
  Gateway In7/1 -> q/1
  Gateway In6/1 -> qv/1
  Gateway Out3/1 -> S-Function/4
  Gateway Out2/1 -> S-Function/3
  Gateway Out1/1 -> S-Function/2
  Gateway Out/1 -> S-Function/1
  S-Function/1 -> Gateway In7/1
  r/1 -> Gateway Out3/1
  w/1 -> Gateway Out2/1
  a/1 -> Gateway Out1/1
  d/1 -> Gateway Out/1
  Gateway Out4/1 -> S-Function/5
  be/1 -> Gateway Out4/1

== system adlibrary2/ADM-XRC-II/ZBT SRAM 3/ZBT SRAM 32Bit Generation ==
  d : Inport  Port=1  LatchInput=off
  a : Inport  Port=2  LatchInput=off
  w : Inport  Port=3  LatchInput=off
  r : Inport  Port=4  LatchInput=off
  be : Inport  Port=5  LatchInput=off
  Black Box : xbsIndex_r3/Black Box  init_code=zbt32_config  sim_method=Inactive  show_param=on
  Constant : Constant  Value=0
  Terminator{,1..3} (4 alike) : Terminator
  ra3 : xbsIndex_r3/Gateway Out  hdl_port=on  timing_constraint=None  locs_specified=off  LOCs={}  needs_fixed_name=off  show_param=off
  rc3 : xbsIndex_r3/Gateway Out  hdl_port=on  timing_constraint=None  locs_specified=off  LOCs={}  needs_fixed_name=off  show_param=off
  rd3_i : xbsIndex_r3/Gateway In  arith_type=Unsigned  n_bits=32  bin_pt=0  quantization=Truncate  overflow=Wrap  period=1  timing_constraint=None  locs_specified=off  LOCs={}  needs_fixed_name=off  dbl_ovrd=off  show_param=off
  rd3_o : xbsIndex_r3/Gateway Out  hdl_port=on  timing_constraint=None  locs_specified=off  LOCs={}  needs_fixed_name=off  show_param=off
  rd3_t : xbsIndex_r3/Gateway Out  hdl_port=on  timing_constraint=None  locs_specified=off  LOCs={}  needs_fixed_name=off  show_param=off
  q : Outport
  qv : Outport  Port=2
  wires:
  Black Box/6 -> rc3/1
  Black Box/5 -> ra3/1
  Black Box/4 -> rd3_t/1
  Black Box/3 -> rd3_o/1
  r/1 -> Black Box/4
  w/1 -> Black Box/3
  a/1 -> Black Box/2
  rc3/1 -> Terminator3/1
  ra3/1 -> Terminator2/1
  rd3_t/1 -> Terminator1/1
  rd3_o/1 -> Terminator/1
  Constant/1 -> rd3_i/1
  Black Box/2 -> qv/1
  Black Box/1 -> q/1
  d/1 -> Black Box/1
  rd3_i/1 -> Black Box/6
  be/1 -> Black Box/5

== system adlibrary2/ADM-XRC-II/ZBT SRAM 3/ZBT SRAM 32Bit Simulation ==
  d : Inport  Port=1  LatchInput=off
  a : Inport  Port=2  LatchInput=off
  w : Inport  Port=3  LatchInput=off
  r : Inport  Port=4  LatchInput=off
  be : Inport  Port=5  LatchInput=off
  Disregard Subsystem : xbsIndex_r3/Disregard Subsystem  Tag=discardX
  Gateway In6 : xbsIndex_r3/Gateway In  arith_type=Boolean  n_bits=1  bin_pt=0  quantization=Truncate  overflow=Wrap  period=1  timing_constraint=None  locs_specified=off  LOCs={}  needs_fixed_name=off  dbl_ovrd=on  show_param=off
  Gateway In7 : xbsIndex_r3/Gateway In  arith_type=Unsigned  n_bits=32  bin_pt=0  quantization=Truncate  overflow=Wrap  period=1  timing_constraint=None  locs_specified=off  LOCs={}  needs_fixed_name=off  dbl_ovrd=on  show_param=off
  Gateway Out{,1..4} (5 alike) : xbsIndex_r3/Gateway Out  hdl_port=off  timing_constraint=None  locs_specified=off  LOCs={}  needs_fixed_name=off  show_param=off
  S-Function : S-Function  FunctionName=zbt32
  q : Outport
  qv : Outport  Port=2
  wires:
  S-Function/2 -> Gateway In6/1
  Gateway In7/1 -> q/1
  Gateway In6/1 -> qv/1
  Gateway Out3/1 -> S-Function/4
  Gateway Out2/1 -> S-Function/3
  Gateway Out1/1 -> S-Function/2
  Gateway Out/1 -> S-Function/1
  S-Function/1 -> Gateway In7/1
  r/1 -> Gateway Out3/1
  w/1 -> Gateway Out2/1
  a/1 -> Gateway Out1/1
  d/1 -> Gateway Out/1
  Gateway Out4/1 -> S-Function/5
  be/1 -> Gateway Out4/1

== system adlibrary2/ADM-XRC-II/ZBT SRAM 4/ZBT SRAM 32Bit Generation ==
  d : Inport  Port=1  LatchInput=off
  a : Inport  Port=2  LatchInput=off
  w : Inport  Port=3  LatchInput=off
  r : Inport  Port=4  LatchInput=off
  be : Inport  Port=5  LatchInput=off
  Black Box : xbsIndex_r3/Black Box  init_code=zbt32_config  sim_method=Inactive  show_param=on
  Constant : Constant  Value=0
  Terminator{,1..3} (4 alike) : Terminator
  ra4 : xbsIndex_r3/Gateway Out  hdl_port=on  timing_constraint=None  locs_specified=off  LOCs={}  needs_fixed_name=off  show_param=off
  rc4 : xbsIndex_r3/Gateway Out  hdl_port=on  timing_constraint=None  locs_specified=off  LOCs={}  needs_fixed_name=off  show_param=off
  rd4_i : xbsIndex_r3/Gateway In  arith_type=Unsigned  n_bits=32  bin_pt=0  quantization=Truncate  overflow=Wrap  period=1  timing_constraint=None  locs_specified=off  LOCs={}  needs_fixed_name=off  dbl_ovrd=off  show_param=off
  rd4_o : xbsIndex_r3/Gateway Out  hdl_port=on  timing_constraint=None  locs_specified=off  LOCs={}  needs_fixed_name=off  show_param=off
  rd4_t : xbsIndex_r3/Gateway Out  hdl_port=on  timing_constraint=None  locs_specified=off  LOCs={}  needs_fixed_name=off  show_param=off
  q : Outport
  qv : Outport  Port=2
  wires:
  Black Box/6 -> rc4/1
  Black Box/5 -> ra4/1
  Black Box/4 -> rd4_t/1
  Black Box/3 -> rd4_o/1
  r/1 -> Black Box/4
  w/1 -> Black Box/3
  a/1 -> Black Box/2
  rc4/1 -> Terminator3/1
  ra4/1 -> Terminator2/1
  rd4_t/1 -> Terminator1/1
  rd4_o/1 -> Terminator/1
  Constant/1 -> rd4_i/1
  Black Box/2 -> qv/1
  Black Box/1 -> q/1
  d/1 -> Black Box/1
  rd4_i/1 -> Black Box/6
  be/1 -> Black Box/5

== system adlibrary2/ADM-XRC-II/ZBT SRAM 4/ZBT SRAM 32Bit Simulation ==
  d : Inport  Port=1  LatchInput=off
  a : Inport  Port=2  LatchInput=off
  w : Inport  Port=3  LatchInput=off
  r : Inport  Port=4  LatchInput=off
  be : Inport  Port=5  LatchInput=off
  Disregard Subsystem : xbsIndex_r3/Disregard Subsystem  Tag=discardX
  Gateway In6 : xbsIndex_r3/Gateway In  arith_type=Boolean  n_bits=1  bin_pt=0  quantization=Truncate  overflow=Wrap  period=1  timing_constraint=None  locs_specified=off  LOCs={}  needs_fixed_name=off  dbl_ovrd=on  show_param=off
  Gateway In7 : xbsIndex_r3/Gateway In  arith_type=Unsigned  n_bits=32  bin_pt=0  quantization=Truncate  overflow=Wrap  period=1  timing_constraint=None  locs_specified=off  LOCs={}  needs_fixed_name=off  dbl_ovrd=on  show_param=off
  Gateway Out{,1..4} (5 alike) : xbsIndex_r3/Gateway Out  hdl_port=off  timing_constraint=None  locs_specified=off  LOCs={}  needs_fixed_name=off  show_param=off
  S-Function : S-Function  FunctionName=zbt32
  q : Outport
  qv : Outport  Port=2
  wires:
  S-Function/2 -> Gateway In6/1
  Gateway In7/1 -> q/1
  Gateway In6/1 -> qv/1
  Gateway Out3/1 -> S-Function/4
  Gateway Out2/1 -> S-Function/3
  Gateway Out1/1 -> S-Function/2
  Gateway Out/1 -> S-Function/1
  S-Function/1 -> Gateway In7/1
  r/1 -> Gateway Out3/1
  w/1 -> Gateway Out2/1
  a/1 -> Gateway Out1/1
  d/1 -> Gateway Out/1
  Gateway Out4/1 -> S-Function/5
  be/1 -> Gateway Out4/1

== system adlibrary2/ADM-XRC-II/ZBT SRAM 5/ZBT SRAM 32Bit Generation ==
  d : Inport  Port=1  LatchInput=off
  a : Inport  Port=2  LatchInput=off
  w : Inport  Port=3  LatchInput=off
  r : Inport  Port=4  LatchInput=off
  be : Inport  Port=5  LatchInput=off
  Black Box : xbsIndex_r3/Black Box  init_code=zbt32_config  sim_method=Inactive  show_param=on
  Constant : Constant  Value=0
  Terminator{,1..3} (4 alike) : Terminator
  ra5 : xbsIndex_r3/Gateway Out  hdl_port=on  timing_constraint=None  locs_specified=off  LOCs={}  needs_fixed_name=off  show_param=off
  rc5 : xbsIndex_r3/Gateway Out  hdl_port=on  timing_constraint=None  locs_specified=off  LOCs={}  needs_fixed_name=off  show_param=off
  rd5_i : xbsIndex_r3/Gateway In  arith_type=Unsigned  n_bits=32  bin_pt=0  quantization=Truncate  overflow=Wrap  period=1  timing_constraint=None  locs_specified=off  LOCs={}  needs_fixed_name=off  dbl_ovrd=off  show_param=off
  rd5_o : xbsIndex_r3/Gateway Out  hdl_port=on  timing_constraint=None  locs_specified=off  LOCs={}  needs_fixed_name=off  show_param=off
  rd5_t : xbsIndex_r3/Gateway Out  hdl_port=on  timing_constraint=None  locs_specified=off  LOCs={}  needs_fixed_name=off  show_param=off
  q : Outport
  qv : Outport  Port=2
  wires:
  Black Box/6 -> rc5/1
  Black Box/5 -> ra5/1
  Black Box/4 -> rd5_t/1
  Black Box/3 -> rd5_o/1
  r/1 -> Black Box/4
  w/1 -> Black Box/3
  a/1 -> Black Box/2
  rc5/1 -> Terminator3/1
  ra5/1 -> Terminator2/1
  rd5_t/1 -> Terminator1/1
  rd5_o/1 -> Terminator/1
  Constant/1 -> rd5_i/1
  Black Box/2 -> qv/1
  Black Box/1 -> q/1
  d/1 -> Black Box/1
  rd5_i/1 -> Black Box/6
  be/1 -> Black Box/5
